{attribute 'qualified_only'}
FUNCTION_BLOCK FB_BaseNode IMPLEMENTS I_TreeNode, I_Errorable
VAR
    eLastStatus : E_NodeStatus := E_NodeStatus.IDLE;
    _sNodeName : STRING(50);
    rProgress : REAL := 0.0;
    _fbErrorHandler : FB_ErrorHandler;
    _sFailedChildName : STRING(50);
    _ipParent : I_TreeNode;
    _bHalted : BOOL := FALSE;
END_VAR

PROPERTY NodeName : STRING(50)
GET
NodeName := _sNodeName;
END_GET
SET
_sNodeName := NodeName;
_fbErrorHandler.Initialize(_sNodeName);
END_SET
END_PROPERTY

METHOD Tick : E_NodeStatus
Tick := E_NodeStatus.IDLE;
END_METHOD

METHOD Halt
_bHalted := TRUE;
eLastStatus := E_NodeStatus.IDLE;
rProgress := 0.0;
END_METHOD

METHOD Reset : BOOL
_bHalted := FALSE;
eLastStatus := E_NodeStatus.IDLE;
rProgress := 0.0;
ClearError();
Reset := TRUE;
END_METHOD

METHOD PUBLIC HasError : BOOL
HasError := _fbErrorHandler.IsActive();
END_METHOD

METHOD PUBLIC GetError : ST_Error
GetError := _fbErrorHandler.GetError();
END_METHOD

METHOD PUBLIC ClearError
_fbErrorHandler.Clear();
_sFailedChildName := '';
END_METHOD

METHOD PUBLIC GetProgress : REAL
GetProgress := rProgress;
END_METHOD

END_FUNCTION_BLOCK
